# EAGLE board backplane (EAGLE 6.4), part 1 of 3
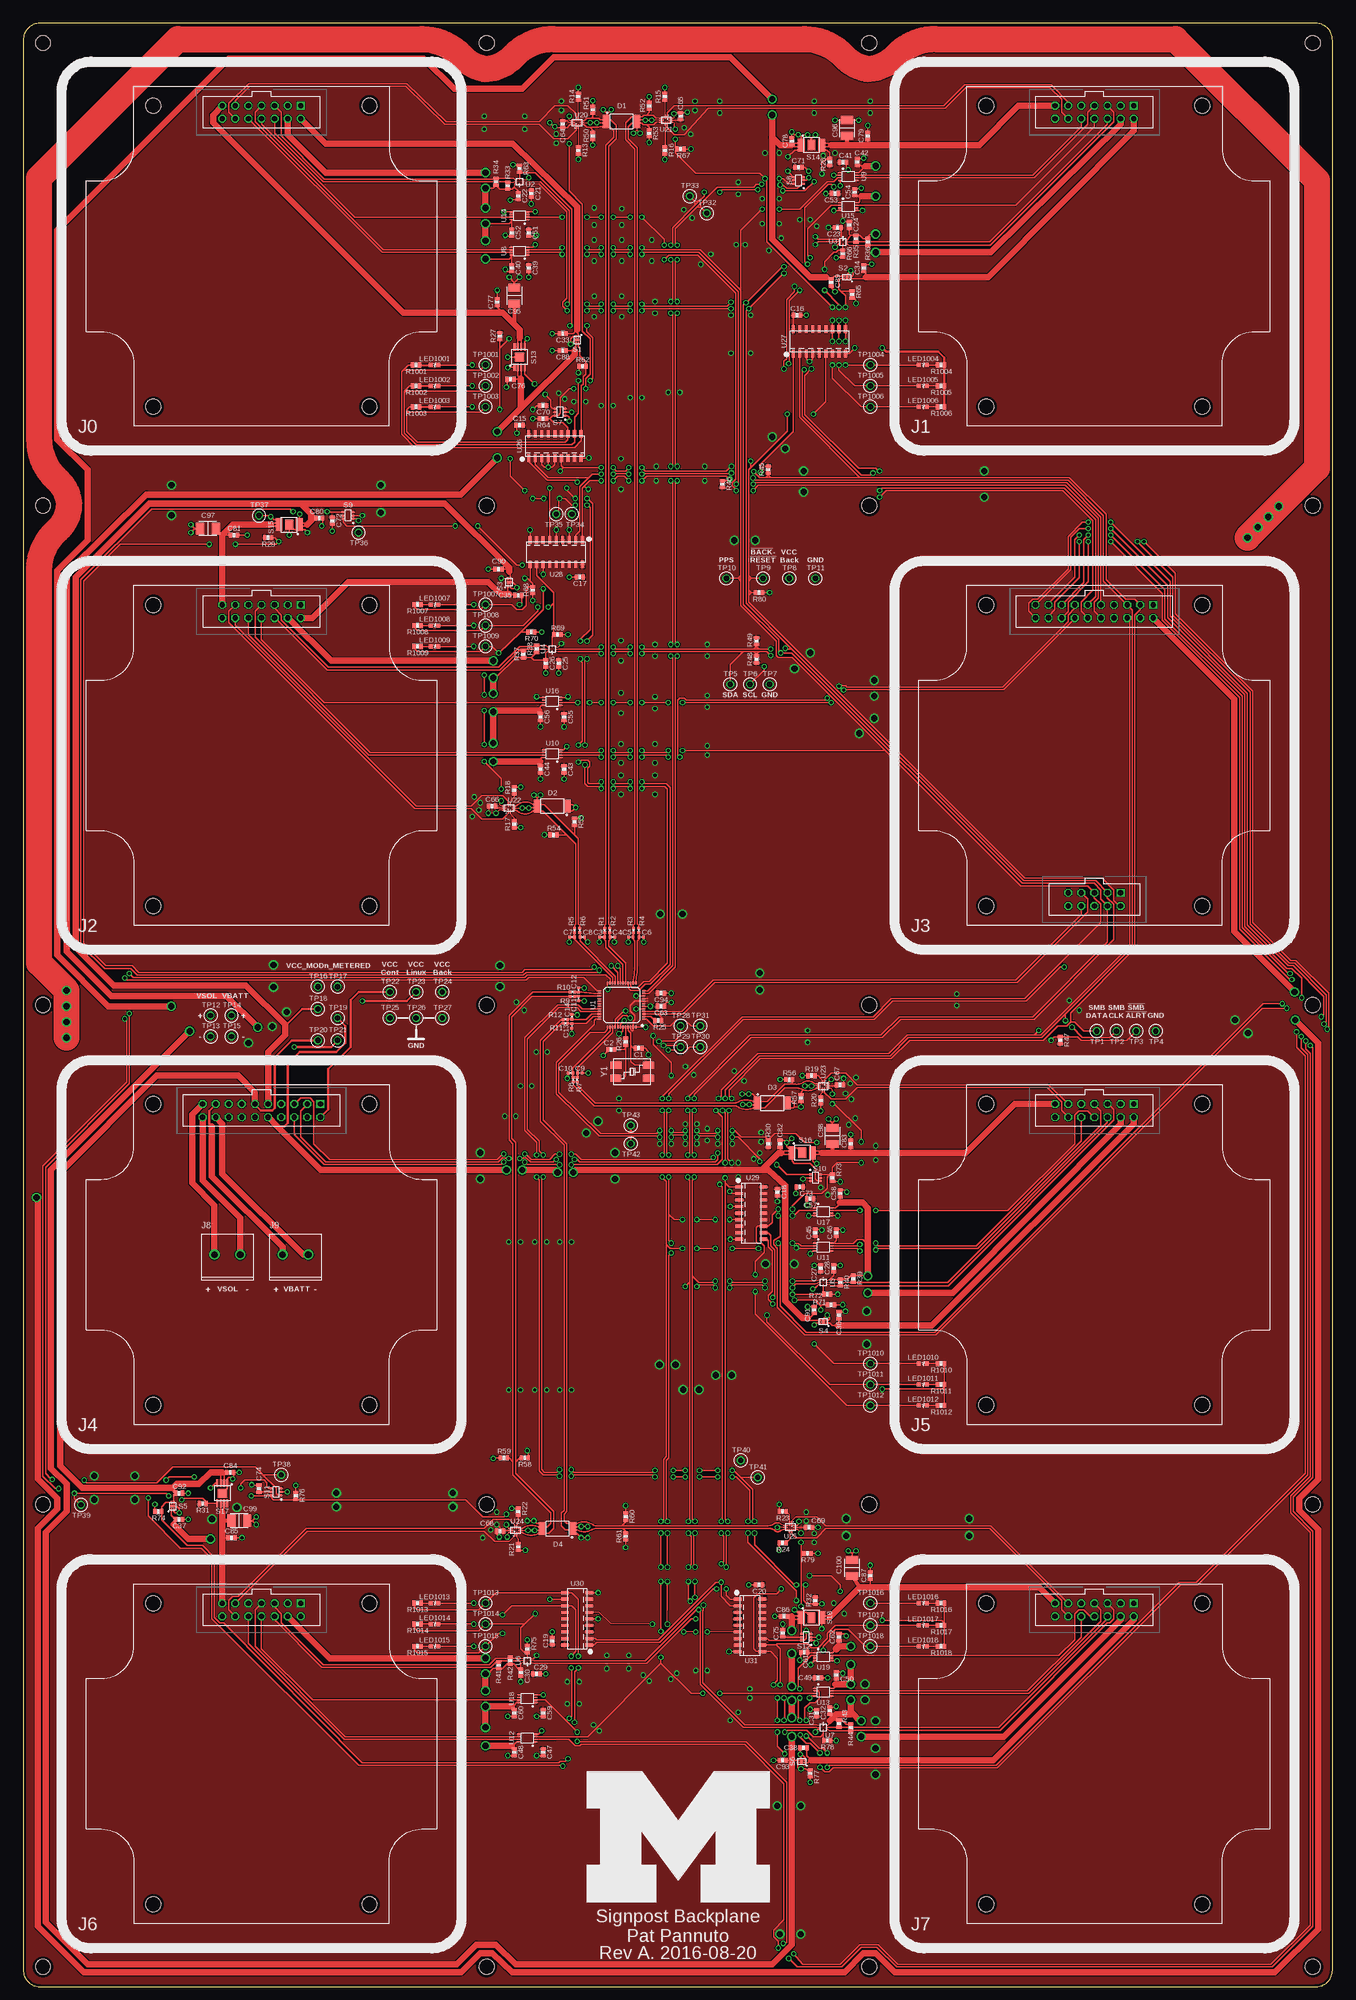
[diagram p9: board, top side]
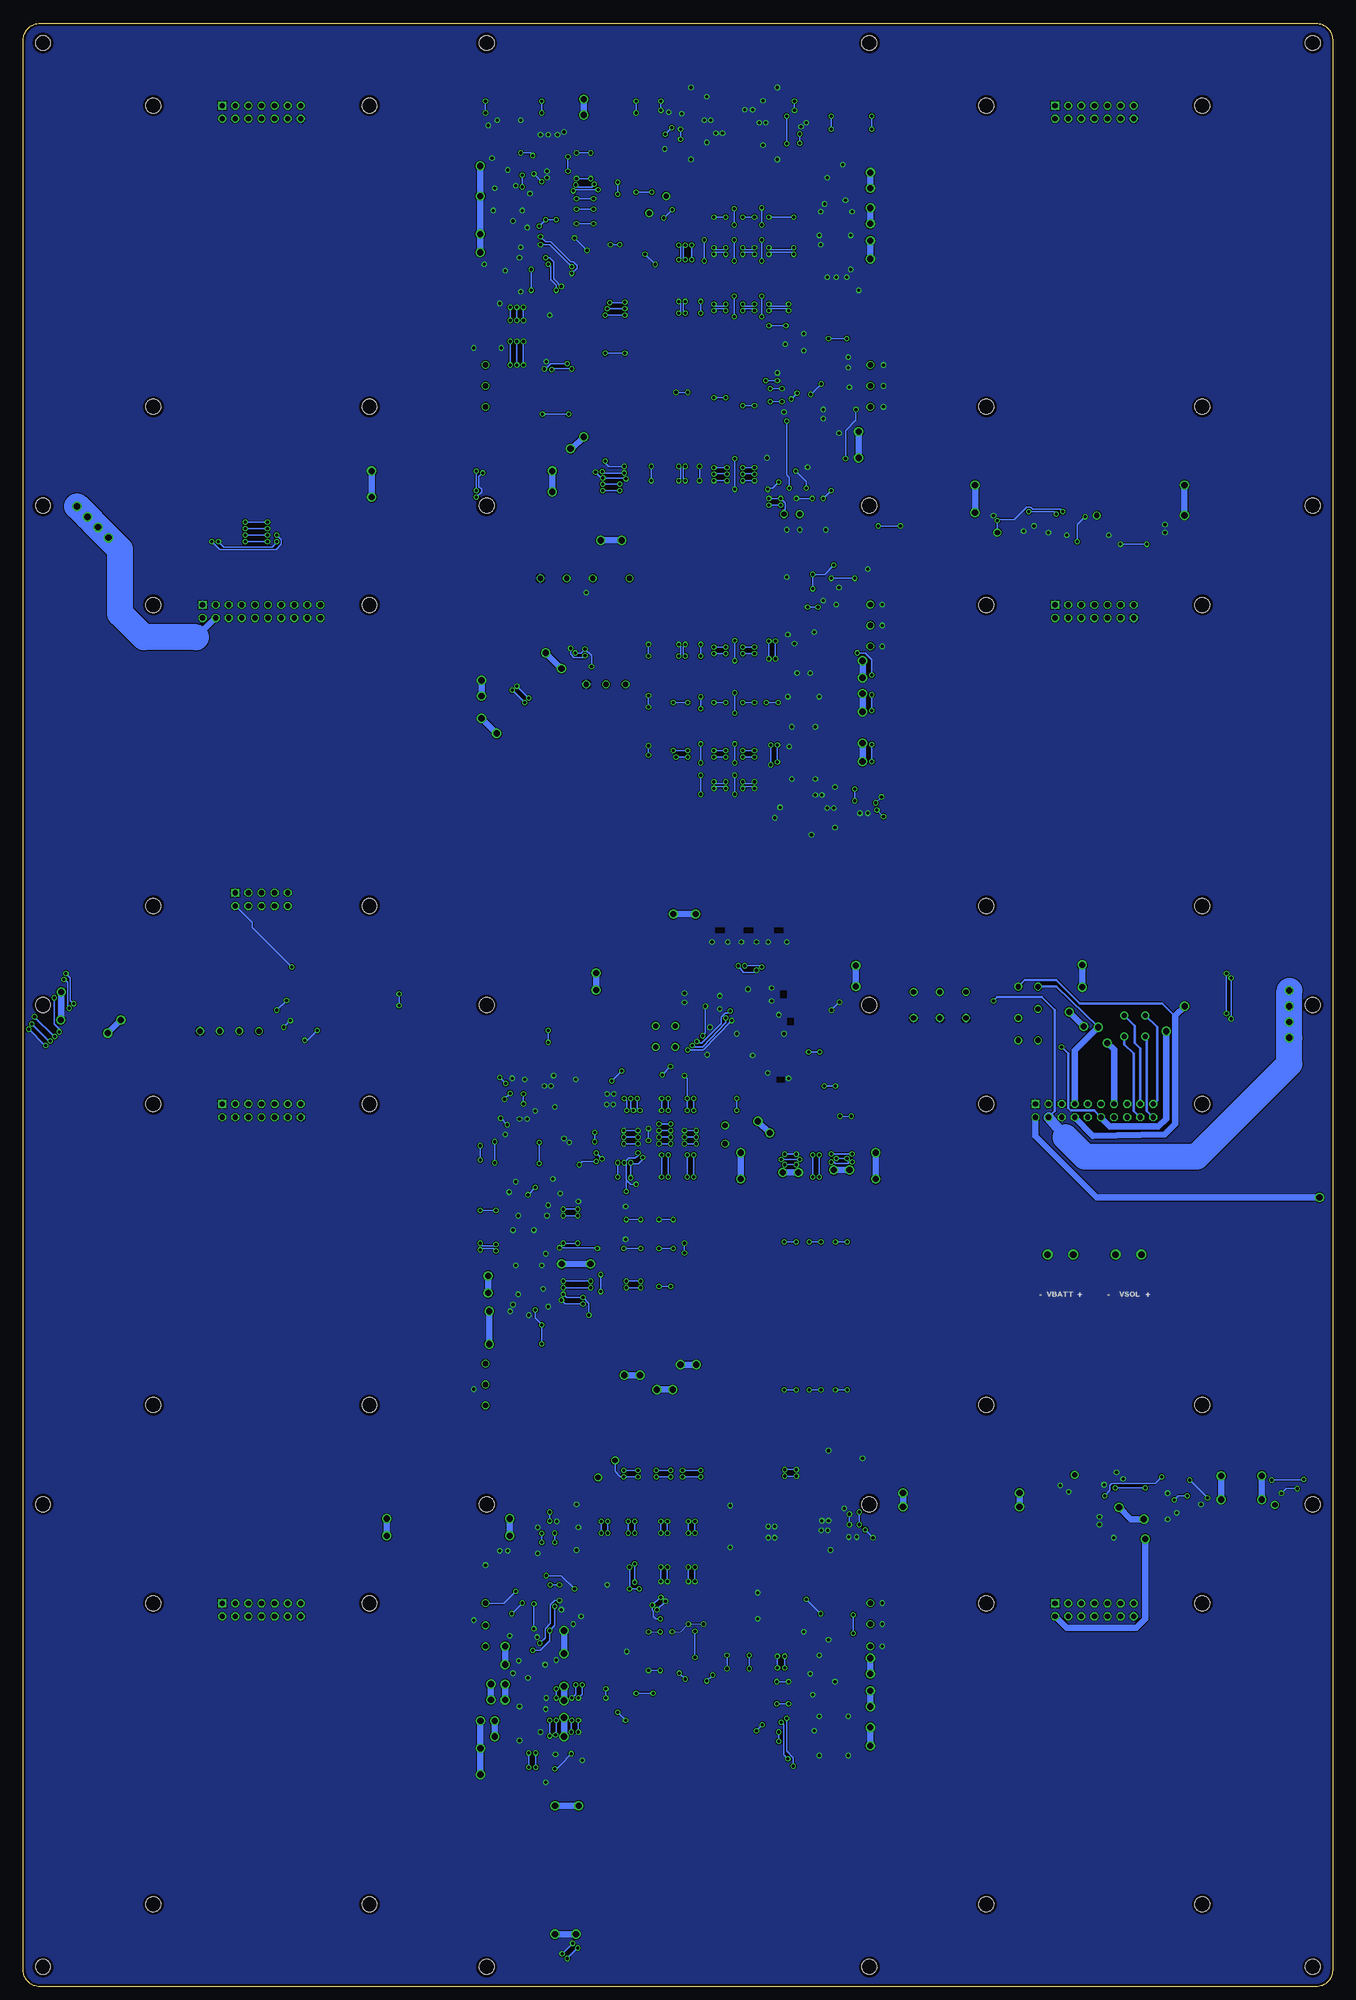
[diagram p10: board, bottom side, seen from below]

Size 254 x 381 mm. Coordinates in mm from the lower left corner, seen from the top.
Outline: 0,377.82 0,3.17 arc90 3.17,0 250.82,0 arc90 254,3.17 254,377.76 arc90 250.76,381 3.17,381 arc90 0,377.82
Copper layers (1*16): Top 0.0178mm / dielectric 59mil / Bottom 0.0178mm
Design rules "sunstone-2lyr_v1.0.0.3 *": minimum track width 6mil, minimum drill 14mil, track to track 6mil, track to pad 6mil, pad to pad 6mil, via to via 6mil, smd to smd 6mil, copper to edge 20mil, drill to drill 16mil, minimum pad ring 8mil, minimum via ring 8mil, stop-mask expansion 3mil, vias tented up to drill 50mil, thermal gap 10mil
Holes 2.95 mm at 3.81,3.81 250.19,3.81 250.19,377.19 3.81,377.19 89.87,377.19 164.13,377.19 3.81,287.38 89.87,287.38 164.13,287.38 250.19,287.38 3.81,190.5 89.87,190.5 164.13,190.5 250.19,190.5 3.81,93.62 89.87,93.62 164.13,93.62 250.19,93.62 89.87,3.81 164.13,3.81
tRestrict: area 120.2,191.5 to 120.5,191.5; area 118,186.1 to 118.1,186.4

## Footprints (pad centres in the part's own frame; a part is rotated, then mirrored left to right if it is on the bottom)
0603_CAP = smd 0.7 x 1: 1 -0.65,0; 2 0.65,0
0402_CAP = smd 0.536 x 0.546: 1 -0.433,0; 2 0.433,0
1210_CAP = smd 2.4 x 1.6: 1 0,1.55; 2 0,-1.55
TSSOP-8 = smd 1.5 x 0.45: 1 -2.9,0.975; 2 -2.9,0.325; 3 -2.9,-0.325; 4 -2.9,-0.975; 5 2.9,-0.975; 6 2.9,-0.325; 7 2.9,0.325; 8 2.9,0.975
BACKPLANE_MODULE_14PIN = drill 1.016 square: 1 7.62,29.21 | drill 1.016 octagon: 2 7.62,26.67; 3 5.08,29.21; 4 5.08,26.67; 5 2.54,29.21; 6 2.54,26.67; 7 0,29.21; 8 0,26.67; 9 -2.54,29.21; 10 -2.54,26.67; 11 -5.08,29.21; 12 -5.08,26.67; 13 -7.62,29.21; 14 -7.62,26.67 | hole 2.946: -20.955,29.21; 20.955,29.21; 20.955,-29.21; -20.955,-29.21
BACKPLANE_MODULE_20PIN_10PIN = drill 1.016 square: 1 11.43,29.21; 21 5.08,-26.67 | drill 1.016 octagon: 2 11.43,26.67; 3 8.89,29.21; 4 8.89,26.67; 5 6.35,29.21; 6 6.35,26.67; 7 3.81,29.21; 8 3.81,26.67; 9 1.27,29.21; 10 1.27,26.67; 11 -1.27,29.21; 12 -1.27,26.67; 13 -3.81,29.21; 14 -3.81,26.67; 15 -6.35,29.21; 16 -6.35,26.67; 17 -8.89,29.21; 18 -8.89,26.67; 19 -11.43,29.21; 20 -11.43,26.67; 22 5.08,-29.21; 23 2.54,-26.67; 24 2.54,-29.21; 25 0,-26.67; 26 0,-29.21; 27 -2.54,-26.67; 28 -2.54,-29.21; 29 -5.08,-26.67; 30 -5.08,-29.21 | hole 2.946: -20.955,29.21; 20.955,29.21; 20.955,-29.21; -20.955,-29.21
BACKPLANE_MODULE_20PIN = drill 1.016 square: 1 11.43,29.21 | drill 1.016 octagon: 2 11.43,26.67; 3 8.89,29.21; 4 8.89,26.67; 5 6.35,29.21; 6 6.35,26.67; 7 3.81,29.21; 8 3.81,26.67; 9 1.27,29.21; 10 1.27,26.67; 11 -1.27,29.21; 12 -1.27,26.67; 13 -3.81,29.21; 14 -3.81,26.67; 15 -6.35,29.21; 16 -6.35,26.67; 17 -8.89,29.21; 18 -8.89,26.67; 19 -11.43,29.21; 20 -11.43,26.67 | hole 2.946: -20.955,29.21; 20.955,29.21; 20.955,-29.21; -20.955,-29.21
PHEONIX-1935161 = drill 1.3: 1 0,0; 2 5,0
LED-0603 = smd 0.8 x 0.8: A 0,-0.75; C 0,0.75
0402_RES-HIGH_SPEED = smd 0.536 x 0.546: 1 -0.433,0; 2 0.433,0
0603-RES = smd 0.7 x 1: 1 -0.65,0; 2 0.65,0
TDFN4 = smd 0.3 x 0.55: 1 -0.25,-0.725; 2 0.25,-0.725; 3 0.25,0.725; 4 -0.25,0.725 | smd 0.86 x 0.5: PAD 0,0
SC70-6 = smd 0.4 x 0.5: 1 -0.65,-0.95; 2 0,-0.95; 3 0.65,-0.95; 4 0.65,0.95; 5 0,0.95; 6 -0.65,0.95
MSOP-8EP = smd 0.45 x 1.35: 1 -0.975,-1.975; 2 -0.325,-1.975; 3 0.325,-1.975; 4 0.975,-1.975; 5 0.975,1.975; 6 0.325,1.975; 7 -0.325,1.975; 8 -0.975,1.975 | smd 2 x 1.7: PAD 0,0
TESTPOINT_0.040IN = drill 1.016: TESTPOINT 0,0
LQFP-48 = smd 0.3 x 0.6: 1 -2.75,-4.3; 2 -2.25,-4.3; 3 -1.75,-4.3; 4 -1.25,-4.3; 5 -0.75,-4.3; 6 -0.25,-4.3; 7 0.25,-4.3; 8 0.75,-4.3; 9 1.25,-4.3; 10 1.75,-4.3; 11 2.25,-4.3; 12 2.75,-4.3; 25 2.75,4.3; 26 2.25,4.3; 27 1.75,4.3; 28 1.25,4.3; 29 0.75,4.3; 30 0.25,4.3; 31 -0.25,4.3; 32 -0.75,4.3; 33 -1.25,4.3; 34 -1.75,4.3; 35 -2.25,4.3; 36 -2.75,4.3 | smd 0.6 x 0.3: 13 4.3,-2.75; 14 4.3,-2.25; 15 4.3,-1.75; 16 4.3,-1.25; 17 4.3,-0.75; 18 4.3,-0.25; 19 4.3,0.25; 20 4.3,0.75; 21 4.3,1.25; 22 4.3,1.75; 23 4.3,2.25; 24 4.3,2.75; 37 -4.3,2.75; 38 -4.3,2.25; 39 -4.3,1.75; 40 -4.3,1.25; 41 -4.3,0.75; 42 -4.3,0.25; 43 -4.3,-0.25; 44 -4.3,-0.75; 45 -4.3,-1.25; 46 -4.3,-1.75; 47 -4.3,-2.25; 48 -4.3,-2.75
UMLP-8 = smd 0.35 x 0.25: 1 -0.55,0; 5 0.55,0 | smd 0.24 x 0.35: 2 -0.4,-0.625; 3 0,-0.625; 4 0.4,-0.625; 6 0.4,0.625; 7 0,0.625; 8 -0.4,0.625
VFSOP-8 = smd 0.25 x 0.75: 1 -0.75,-1.55; 2 -0.25,-1.55; 3 0.25,-1.55; 4 0.75,-1.55; 5 0.75,1.55; 6 0.25,1.55; 7 -0.25,1.55; 8 -0.75,1.55
UQFN-10 = smd 0.2 x 0.9: 1 -0.2,-0.65 | smd 0.2 x 0.8: 2 0.2,-0.7; 6 0.2,0.7; 7 -0.2,0.7 | smd 0.8 x 0.2: 3 0.9,-0.4; 4 0.9,0; 5 0.9,0.4; 8 -0.9,0.4; 9 -0.9,0; 10 -0.9,-0.4
SOIC-18 = smd 0.635 x 1.524: 1 -5.08,-2.362; 2 -3.81,-2.362; 3 -2.54,-2.362; 4 -1.27,-2.362; 5 0,-2.362; 6 1.27,-2.362; 7 2.54,-2.362; 8 3.81,-2.362; 9 5.08,-2.362; 10 5.08,2.362; 11 3.81,2.362; 12 2.54,2.362; 13 1.27,2.362; 14 0,2.362; 15 -1.27,2.362; 16 -2.54,2.362; 17 -3.81,2.362; 18 -5.08,2.362
ABMM = smd 2.21 x 1.397: 1 -3.167,-1.27; 3 3.15,1.27; NC1 -3.15,1.27; NC2 3.15,-1.27

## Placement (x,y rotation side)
C1  22pF, 5% tol  [0603_CAP]  119.38,182.12 180 top
C2  22pF, 5% tol  [0603_CAP]  114.05,181.86 0 top
C3  22pF  [0402_CAP]  112.27,203.71 180 top
C4  22pF  [0402_CAP]  114.3,203.71 0 top
C5  22pF  [0402_CAP]  117.86,203.71 180 top
C6  22pF  [0402_CAP]  119.89,203.71 0 top
C7  22pF  [0402_CAP]  106.43,203.71 180 top
C8  22pF  [0402_CAP]  108.46,203.71 0 top
C9  22pF  [0402_CAP]  107.95,177.29 0 top
C10  22pF  [0402_CAP]  106.17,177.29 180 top
C11  22pF  [0402_CAP]  107.7,191.77 270 top
C12  22pF  [0402_CAP]  107.7,193.42 90 top
C13  22pF  [0402_CAP]  106.43,186.44 270 top
C14  22pF  [0402_CAP]  106.43,188.21 90 top
C15  100nF  [0603_CAP]  96.27,303.02 180 top
C16  100nF  [0603_CAP]  150.11,324.36 0 top
C17  100nF  [0603_CAP]  107.95,273.56 180 top
C18  100nF  [0603_CAP]  146.3,154.18 270 top
C19  100nF  [0603_CAP]  102.62,67.06 90 top
C20  100nF  [0603_CAP]  142.75,77.98 180 top
C21  100nF  [0603_CAP]  98.55,347.98 270 top
C22  100nF  [0603_CAP]  96.01,347.47 270 top
C23  100nF  [0603_CAP]  157.99,341.38 180 top
C24  100nF  [0603_CAP]  160.27,341.88 90 top
C25  100nF  [0603_CAP]  103.89,256.79 270 top
C26  100nF  [0603_CAP]  101.35,256.79 270 top
C27  100nF  [0603_CAP]  154.69,139.45 90 top
C28  100nF  [0603_CAP]  157.23,139.45 90 top
C29  100nF  [0603_CAP]  99.57,60.71 0 top
C30  100nF  [0603_CAP]  96.52,60.96 270 top
C31  100nF  [0603_CAP]  153.92,53.09 90 top
C32  100nF  [0603_CAP]  156.46,53.59 90 top
C33  100nF  [0603_CAP]  104.65,320.8 180 top
C34  100nF  [0603_CAP]  163.07,333.5 90 top
C35  100nF  [0603_CAP]  96.01,270 0 top
C36  100nF  [0603_CAP]  158.24,130.3 90 top
C37  100nF  [0603_CAP]  30.23,90.68 0 top
C38  100nF  [0603_CAP]  151.38,46.35 180 top
C39  100nF  [0603_CAP]  98.04,333.5 270 top
C40  100nF  [0603_CAP]  94.74,333.5 270 top
C41  100nF  [0603_CAP]  159,354.08 0 top
C42  100nF  [0603_CAP]  161.8,354.08 90 top
C43  100nF  [0603_CAP]  104.9,236.22 270 top
C44  100nF  [0603_CAP]  100.33,236.22 270 top
C45  100nF  [0603_CAP]  153.67,146.3 90 top
C46  100nF  [0603_CAP]  157.73,146.3 90 top
C47  100nF  [0603_CAP]  100.84,45.47 270 top
C48  100nF  [0603_CAP]  95.25,45.47 270 top
C49  100nF  [0603_CAP]  154.18,59.94 0 top
C50  100nF  [0603_CAP]  157.73,60.45 90 top
C51  100nF  [0603_CAP]  98.04,340.36 270 top
C52  100nF  [0603_CAP]  94.74,340.36 270 top
C53  100nF  [0603_CAP]  157.48,347.98 180 top
C54  100nF  [0603_CAP]  161.29,348.23 90 top
C55  100nF  [0603_CAP]  104.9,246.38 270 top
C56  100nF  [0603_CAP]  100.33,246.38 270 top
C57  100nF  [0603_CAP]  152.65,152.91 180 top
C58  100nF  [0603_CAP]  158.5,153.92 90 top
C59  100nF  [0603_CAP]  100.84,53.09 270 top
C60  100nF  [0603_CAP]  95.25,53.09 270 top
C61  100nF  [0603_CAP]  151.51,64.9 180 top
C62  100nF  [0603_CAP]  158.24,67.82 90 top
C63  100nF  [0603_CAP]  123.7,190.25 180 top
C64  100nF  [0603_CAP]  104.65,361.44 90 top
C65  100nF  [0603_CAP]  127.51,362.97 270 top
C66  100nF  [0603_CAP]  90.93,229.11 0 top
C67  100nF  [0603_CAP]  158.47,175.01 180 top
C68  100nF  [0603_CAP]  92.46,88.39 0 top
C69  100nF  [0603_CAP]  152.4,89.15 180 top
C70  100nF  [0603_CAP]  100.84,306.83 180 top
C71  100nF  [0603_CAP]  150.37,353.06 0 top
C72  100nF  [0603_CAP]  59.94,284.48 270 top
C73  100nF  [0603_CAP]  150.62,155.19 180 top
C74  100nF  [0603_CAP]  45.72,96.65 90 top
C75  100nF  [0603_CAP]  147.32,68.58 90 top
C76  100nF  [0603_CAP]  94.49,311.91 180 top
C77  100nF  [0603_CAP]  91.95,326.9 90 top
C78  100nF  [0603_CAP]  149.1,358.14 90 top
C79  100nF  [0603_CAP]  163.83,359.16 90 top
C80  100nF  [0603_CAP]  57.4,284.99 0 top
C81  100nF  [0603_CAP]  40.89,281.69 0 top
C82  100nF  [0603_CAP]  146.81,163.58 90 top
C83  100nF  [0603_CAP]  160.53,163.58 90 top
C84  100nF  [0603_CAP]  40.13,99.82 0 top
C85  100nF  [0603_CAP]  40.39,87.12 0 top
C86  100nF  [0603_CAP]  147.57,71.88 180 top
C87  100nF  [0603_CAP]  164.34,79.76 90 top
C88  4.7uF  [0603_CAP]  104.65,317.5 180 top
C89  4.7uF  [0603_CAP]  156.72,330.71 270 top
C90  4.7uF  [0603_CAP]  92.2,275.08 180 top
C91  4.7uF  [0603_CAP]  153.42,131.32 90 top
C92  4.7uF  [0603_CAP]  30.23,95.76 0 top
C93  4.7uF  [0603_CAP]  147.32,43.94 180 top
C94  4.7uF  [0603_CAP]  123.7,192.79 180 top
C95  150uF  [1210_CAP]  95.25,328.17 180 top
C96  150uF  [1210_CAP]  159.77,360.68 180 top
C97  150uF  [1210_CAP]  35.81,282.96 270 top
C98  150uF  [1210_CAP]  156.97,165.1 180 top
C99  150uF  [1210_CAP]  41.91,90.42 90 top
C100  150uF  [1210_CAP]  160.78,81.28 180 top
D1  SN75240-TSSOP  [TSSOP-8]  116.08,361.95 0 top
D2  SN75240-TSSOP  [TSSOP-8]  102.62,229.11 180 top
D3  SN75240-TSSOP  [TSSOP-8]  145.29,171.45 0 top
D4  SN75240-TSSOP  [TSSOP-8]  103.63,88.9 180 top
J0  BACKPLANE_GENERIC_MODULE  [BACKPLANE_MODULE_14PIN]  46.2,335.81 0 top
J1  BACKPLANE_GENERIC_MODULE  [BACKPLANE_MODULE_14PIN]  207.8,335.81 0 top
J2  BACKPLANE_GENERIC_MODULE  [BACKPLANE_MODULE_14PIN]  46.2,238.94 0 top
J3  BACKPLANE_CONTROLLER_MODULE  [BACKPLANE_MODULE_20PIN_10PIN]  207.8,238.94 0 top
J4  BACKPLANE_POWER_MODULE  [BACKPLANE_MODULE_20PIN]  46.2,142.06 0 top
J5  BACKPLANE_GENERIC_MODULE  [BACKPLANE_MODULE_14PIN]  207.8,142.06 0 top
J6  BACKPLANE_GENERIC_MODULE  [BACKPLANE_MODULE_14PIN]  46.2,45.19 0 top
J7  BACKPLANE_GENERIC_MODULE  [BACKPLANE_MODULE_14PIN]  207.8,45.19 0 top
J8  SCREW_TERMINAL  [PHEONIX-1935161]  37.08,142.06 0 top
J9  SCREW_TERMINAL  [PHEONIX-1935161]  50.29,142.06 0 top
LED1001  LED0603  [LED-0603]  79.76,314.71 270 top
LED1002  LED0603  [LED-0603]  79.76,310.64 270 top
LED1003  LED0603  [LED-0603]  79.76,306.58 270 top
LED1004  LED0603  [LED-0603]  174.5,314.71 270 top
LED1005  LED0603  [LED-0603]  174.5,310.64 270 top
LED1006  LED0603  [LED-0603]  174.5,306.58 270 top
LED1007  LED0603  [LED-0603]  79.76,268.22 270 top
LED1008  LED0603  [LED-0603]  79.76,264.16 270 top
LED1009  LED0603  [LED-0603]  79.76,260.1 270 top
LED1010  LED0603  [LED-0603]  174.5,120.9 270 top
LED1011  LED0603  [LED-0603]  174.5,116.84 270 top
LED1012  LED0603  [LED-0603]  174.5,112.78 270 top
LED1013  LED0603  [LED-0603]  79.76,74.42 270 top
LED1014  LED0603  [LED-0603]  79.76,70.36 270 top
LED1015  LED0603  [LED-0603]  79.76,66.04 270 top
LED1016  LED0603  [LED-0603]  174.5,74.42 270 top
LED1017  LED0603  [LED-0603]  174.5,70.1 270 top
LED1018  LED0603  [LED-0603]  174.5,66.04 270 top
LOGO1  UMICH_SOLID_GIANT  [UMICH_SOLID_1000MIL]  109.35,16.38 0 top
R1  27Ω  [0402_RES-HIGH_SPEED]  112.78,204.98 90 top
R2  27Ω  [0402_RES-HIGH_SPEED]  113.79,204.98 90 top
R3  27Ω  [0402_RES-HIGH_SPEED]  118.36,204.98 90 top
R4  27Ω  [0402_RES-HIGH_SPEED]  119.38,204.98 90 top
R5  27Ω  [0402_RES-HIGH_SPEED]  106.93,204.98 90 top
R6  27Ω  [0402_RES-HIGH_SPEED]  107.95,204.98 90 top
R7  27Ω  [0402_RES-HIGH_SPEED]  107.44,176.02 270 top
R8  27Ω  [0402_RES-HIGH_SPEED]  106.68,176.02 270 top
R9  27Ω  [0402_RES-HIGH_SPEED]  106.55,192.15 180 top
R10  27Ω  [0402_RES-HIGH_SPEED]  106.55,193.04 180 top
R11  27Ω  [0402_RES-HIGH_SPEED]  105.16,186.94 180 top
R12  27Ω  [0402_RES-HIGH_SPEED]  105.16,187.71 180 top
R13  50Ω  [0603-RES]  107.7,356.36 270 top
R14  50Ω  [0603-RES]  107.7,366.78 90 top
R15  50Ω  [0603-RES]  124.46,366.78 90 top
R16  50Ω  [0603-RES]  124.46,356.36 270 top
R17  50Ω  [0603-RES]  95.25,225.55 270 top
R18  50Ω  [0603-RES]  95.25,232.16 90 top
R19  50Ω  [0603-RES]  152.91,176.78 180 top
R20  50Ω  [0603-RES]  154.69,171.96 270 top
R21  50Ω  [0603-RES]  96.01,85.34 270 top
R22  50Ω  [0603-RES]  96.01,92.2 90 top
R23  50Ω  [0603-RES]  147.32,92.2 180 top
R24  50Ω  [0603-RES]  147.32,86.11 180 top
R25  1.5kΩ  [0603-RES]  123.19,187.45 180 top
R26  1.5kΩ  [0603-RES]  116.84,183.39 90 top
R27  10kΩ  [0603-RES]  92.46,320.29 90 top
R28  10kΩ  [0603-RES]  156.46,354.08 270 top
R29  10kΩ  [0603-RES]  47.5,281.18 180 top
R30  10kΩ  [0603-RES]  144.53,163.58 270 top
R31  10kΩ  [0603-RES]  34.8,93.73 180 top
R32  10kΩ  [0603-RES]  153.67,74.93 90 top
R33  10kΩ  [0603-RES]  93.98,349.5 90 top
R34  10kΩ  [0603-RES]  91.69,350.27 90 top
R35  10kΩ  [0603-RES]  161.54,339.22 270 top
R36  10kΩ  [0603-RES]  163.83,338.58 270 top
R37  10kΩ  [0603-RES]  97.03,258.57 90 top
R38  10kΩ  [0603-RES]  99.57,259.59 90 top
R39  10kΩ  [0603-RES]  161.04,137.41 270 top
R40  10kΩ  [0603-RES]  158.5,136.65 270 top
R41  10kΩ  [0603-RES]  92.2,62.36 90 top
R42  10kΩ  [0603-RES]  94.49,63.25 90 top
R43  10kΩ  [0603-RES]  158.24,51.05 270 top
R44  10kΩ  [0603-RES]  160.53,50.29 270 top
R45  10kΩ  [0603-RES]  144.53,294.39 90 top
R46  10kΩ  [0603-RES]  135.64,291.59 270 top
R47  10kΩ  [0603-RES]  201.17,183.64 270 top
R48  10kΩ  [0603-RES]  142.24,257.56 270 top
R49  10kΩ  [0603-RES]  142.24,261.11 90 top
R50  15kΩ  [0603-RES]  110.49,359.16 90 top
R51  15kΩ  [0603-RES]  110.49,364.24 270 top
R52  15kΩ  [0603-RES]  121.41,365 270 top
R53  15kΩ  [0603-RES]  121.41,359.66 90 top
R54  15kΩ  [0603-RES]  102.87,223.52 0 top
R55  15kΩ  [0603-RES]  106.93,226.06 270 top
R56  15kΩ  [0603-RES]  148.59,176.02 0 top
R57  15kΩ  [0603-RES]  150.88,172.47 90 top
R58  15kΩ  [0603-RES]  97.28,102.62 180 top
R59  15kΩ  [0603-RES]  93.22,102.62 0 top
R60  15kΩ  [0603-RES]  116.84,91.19 270 top
R61  15kΩ  [0603-RES]  116.84,87.38 90 top
R62  10MΩ  [0603-RES]  108.46,314.45 0 top
R63  10MΩ  [0603-RES]  96.27,352.81 270 top
R64  10MΩ  [0603-RES]  100.84,304.29 0 top
R65  10MΩ  [0603-RES]  160.78,328.42 90 top
R66  10MΩ  [0603-RES]  159,336.3 90 top
R67  10MΩ  [0603-RES]  127.51,356.62 180 top
R68  10MΩ  [0603-RES]  98.81,271.02 90 top
R69  10MΩ  [0603-RES]  103.63,262.38 180 top
R70  10MΩ  [0603-RES]  98.55,262.89 180 top
R71  10MΩ  [0603-RES]  156.72,132.33 180 top
R72  10MΩ  [0603-RES]  155.96,134.37 180 top
R73  10MΩ  [0603-RES]  156.97,156.97 90 top
R74  10MΩ  [0603-RES]  26.16,92.2 0 top
R75  10MΩ  [0603-RES]  97.79,65.53 270 top
R76  10MΩ  [0603-RES]  52.83,95.25 270 top
R77  10MΩ  [0603-RES]  152.65,41.4 90 top
R78  10MΩ  [0603-RES]  155.96,47.75 180 top
R79  10MΩ  [0603-RES]  152.15,84.07 180 top
R80  10MΩ  [0603-RES]  142.75,270.51 180 top
R1001  15Ω  [0603-RES]  76.2,314.71 180 top
R1002  15Ω  [0603-RES]  76.2,310.64 180 top
R1003  15Ω  [0603-RES]  76.2,306.58 180 top
R1004  15Ω  [0603-RES]  178.05,314.71 180 top
R1005  15Ω  [0603-RES]  178.05,310.64 180 top
R1006  15Ω  [0603-RES]  178.05,306.58 180 top
R1007  15Ω  [0603-RES]  76.45,268.22 180 top
R1008  15Ω  [0603-RES]  76.45,264.16 180 top
R1009  15Ω  [0603-RES]  76.45,260.1 180 top
R1010  15Ω  [0603-RES]  178.05,120.9 180 top
R1011  15Ω  [0603-RES]  178.05,116.84 180 top
R1012  15Ω  [0603-RES]  178.05,112.78 180 top
R1013  15Ω  [0603-RES]  76.45,74.42 180 top
R1014  15Ω  [0603-RES]  76.45,70.36 180 top
R1015  15Ω  [0603-RES]  76.45,66.04 180 top
R1016  15Ω  [0603-RES]  178.05,74.42 180 top
R1017  15Ω  [0603-RES]  178.05,70.1 180 top
R1018  15Ω  [0603-RES]  178.05,66.04 180 top
S1  SIP3240X  [TDFN4]  107.44,319.53 180 top
S2  SIP3240X  [TDFN4]  159.77,331.72 90 top
S3  SIP3240X  [TDFN4]  94.23,272.54 0 top
S4  SIP3240X  [TDFN4]  155.19,129.03 90 top
S5  SIP3240X  [TDFN4]  28.96,93.22 0 top
S6  SIP3240X  [TDFN4]  151,43.69 90 top
S7  NC7SZ157  [SC70-6]  104.14,305.56 90 top
S8  NC7SZ157  [SC70-6]  150.37,350.52 90 top
S9  NC7SZ157  [SC70-6]  62.99,285.5 90 top
S10  NC7SZ157  [SC70-6]  153.67,156.97 270 top
S11  NC7SZ157  [SC70-6]  49.02,96.01 90 top
S12  NC7SZ157  [SC70-6]  151.89,67.82 90 top
S13  AP2401MP  [MSOP-8EP]  96.27,316.23 0 top
S14  AP2401MP  [MSOP-8EP]  152.91,357.38 270 top
S15  AP2401MP  [MSOP-8EP]  51.56,283.72 90 top
S16  AP2401MP  [MSOP-8EP]  151.13,161.8 270 top
S17  AP2401MP  [MSOP-8EP]  38.61,95.76 180 top
S18  AP2401MP  [MSOP-8EP]  152.91,71.63 270 top
TP1  TEST_POINT_0.040IN  [TESTPOINT_0.040IN]  208.28,185.42 0 top
TP2  TEST_POINT_0.040IN  [TESTPOINT_0.040IN]  212.09,185.42 0 top
TP3  TEST_POINT_0.040IN  [TESTPOINT_0.040IN]  215.9,185.42 0 top
TP4  TEST_POINT_0.040IN  [TESTPOINT_0.040IN]  219.71,185.42 0 top
TP5  TEST_POINT_0.040IN  [TESTPOINT_0.040IN]  137.16,252.73 0 top
TP6  TEST_POINT_0.040IN  [TESTPOINT_0.040IN]  140.97,252.73 0 top
TP7  TEST_POINT_0.040IN  [TESTPOINT_0.040IN]  144.78,252.73 0 top
TP8  TEST_POINT_0.040IN  [TESTPOINT_0.040IN]  148.59,273.3 0 top
TP9  TEST_POINT_0.040IN  [TESTPOINT_0.040IN]  143.51,273.3 0 top
TP10  TEST_POINT_0.040IN  [TESTPOINT_0.040IN]  136.4,273.3 0 top
TP11  TEST_POINT_0.040IN  [TESTPOINT_0.040IN]  153.67,273.3 0 top
TP12  TEST_POINT_0.040IN  [TESTPOINT_0.040IN]  36.32,188.47 0 top
TP13  TEST_POINT_0.040IN  [TESTPOINT_0.040IN]  36.32,184.4 0 top
TP14  TEST_POINT_0.040IN  [TESTPOINT_0.040IN]  40.39,188.47 0 top
TP15  TEST_POINT_0.040IN  [TESTPOINT_0.040IN]  40.39,184.4 0 top
TP16  TEST_POINT_0.040IN  [TESTPOINT_0.040IN]  57.15,194.06 0 top
TP17  TEST_POINT_0.040IN  [TESTPOINT_0.040IN]  60.96,194.06 0 top
TP18  TEST_POINT_0.040IN  [TESTPOINT_0.040IN]  57.15,189.74 0 top
TP19  TEST_POINT_0.040IN  [TESTPOINT_0.040IN]  60.96,187.96 0 top
TP20  TEST_POINT_0.040IN  [TESTPOINT_0.040IN]  57.15,183.64 0 top
TP21  TEST_POINT_0.040IN  [TESTPOINT_0.040IN]  60.96,183.64 0 top
TP22  TEST_POINT_0.040IN  [TESTPOINT_0.040IN]  71.12,193.04 0 top
TP23  TEST_POINT_0.040IN  [TESTPOINT_0.040IN]  76.2,193.04 0 top
TP24  TEST_POINT_0.040IN  [TESTPOINT_0.040IN]  81.28,193.04 0 top
TP25  TEST_POINT_0.040IN  [TESTPOINT_0.040IN]  71.12,187.96 0 top
TP26  TEST_POINT_0.040IN  [TESTPOINT_0.040IN]  76.2,187.96 0 top
TP27  TEST_POINT_0.040IN  [TESTPOINT_0.040IN]  81.28,187.96 0 top
TP28  TEST_POINT_0.040IN  [TESTPOINT_0.040IN]  127.51,186.44 0 top
TP29  TEST_POINT_0.040IN  [TESTPOINT_0.040IN]  127.51,182.37 0 top
TP30  TEST_POINT_0.040IN  [TESTPOINT_0.040IN]  131.32,182.37 0 top
TP31  TEST_POINT_0.040IN  [TESTPOINT_0.040IN]  131.32,186.44 0 top
TP32  TEST_POINT_0.040IN  [TESTPOINT_0.040IN]  132.59,344.17 0 top
TP33  TEST_POINT_0.040IN  [TESTPOINT_0.040IN]  129.29,347.47 0 top
TP34  TEST_POINT_0.040IN  [TESTPOINT_0.040IN]  106.43,285.75 0 top
TP35  TEST_POINT_0.040IN  [TESTPOINT_0.040IN]  103.38,285.75 0 top
TP36  TEST_POINT_0.040IN  [TESTPOINT_0.040IN]  65.02,282.19 180 top
TP37  TEST_POINT_0.040IN  [TESTPOINT_0.040IN]  45.72,285.5 0 top
TP38  TEST_POINT_0.040IN  [TESTPOINT_0.040IN]  50.04,99.31 0 top
TP39  TEST_POINT_0.040IN  [TESTPOINT_0.040IN]  11.18,93.47 180 top
TP40  TEST_POINT_0.040IN  [TESTPOINT_0.040IN]  139.19,102.11 0 top
TP41  TEST_POINT_0.040IN  [TESTPOINT_0.040IN]  142.49,98.81 0 top
TP42  TEST_POINT_0.040IN  [TESTPOINT_0.040IN]  117.86,163.58 180 top
TP43  TEST_POINT_0.040IN  [TESTPOINT_0.040IN]  117.86,167.13 0 top
TP1001  TEST_POINT_0.040IN  [TESTPOINT_0.040IN]  89.66,314.71 0 top
TP1002  TEST_POINT_0.040IN  [TESTPOINT_0.040IN]  89.66,310.64 0 top
TP1003  TEST_POINT_0.040IN  [TESTPOINT_0.040IN]  89.66,306.58 0 top
TP1004  TEST_POINT_0.040IN  [TESTPOINT_0.040IN]  164.34,314.71 0 top
TP1005  TEST_POINT_0.040IN  [TESTPOINT_0.040IN]  164.34,310.64 0 top
TP1006  TEST_POINT_0.040IN  [TESTPOINT_0.040IN]  164.34,306.58 0 top
TP1007  TEST_POINT_0.040IN  [TESTPOINT_0.040IN]  89.66,268.22 0 top
TP1008  TEST_POINT_0.040IN  [TESTPOINT_0.040IN]  89.66,264.16 0 top
TP1009  TEST_POINT_0.040IN  [TESTPOINT_0.040IN]  89.66,260.1 0 top
TP1010  TEST_POINT_0.040IN  [TESTPOINT_0.040IN]  164.34,120.9 0 top
TP1011  TEST_POINT_0.040IN  [TESTPOINT_0.040IN]  164.34,116.84 0 top
TP1012  TEST_POINT_0.040IN  [TESTPOINT_0.040IN]  164.34,112.78 0 top
TP1013  TEST_POINT_0.040IN  [TESTPOINT_0.040IN]  89.66,74.42 0 top
TP1014  TEST_POINT_0.040IN  [TESTPOINT_0.040IN]  89.66,70.36 0 top
TP1015  TEST_POINT_0.040IN  [TESTPOINT_0.040IN]  89.66,66.04 0 top
TP1016  TEST_POINT_0.040IN  [TESTPOINT_0.040IN]  164.34,74.42 0 top
TP1017  TEST_POINT_0.040IN  [TESTPOINT_0.040IN]  164.34,70.1 0 top
TP1018  TEST_POINT_0.040IN  [TESTPOINT_0.040IN]  164.34,66.04 0 top
U1  TUSB2077A  [LQFP-48]  116.08,190.5 90 top
U2  FXMA2102  [UMLP-8]  96.27,350.27 90 top
U3  FXMA2102  [UMLP-8]  159,338.58 270 top
U4  FXMA2102  [UMLP-8]  102.62,259.59 90 top
U5  FXMA2102  [UMLP-8]  155.19,136.65 270 top
U6  FXMA2102  [UMLP-8]  97.79,63.25 90 top
U7  FXMA2102  [UMLP-8]  155.19,50.29 270 top
U8  SN74LVC2T45  [VFSOP-8]  96.27,336.8 90 top
U9  SN74LVC2T45  [VFSOP-8]  160.02,351.28 270 top
U10  SN74LVC2T45  [VFSOP-8]  102.62,239.27 90 top
U11  SN74LVC2T45  [VFSOP-8]  155.19,143.51 270 top
U12  SN74LVC2T45  [VFSOP-8]  97.79,48.26 90 top
U13  SN74LVC2T45  [VFSOP-8]  155.19,57.15 270 top
U14  SN74LVC2T45  [VFSOP-8]  96.27,343.66 90 top
U15  SN74LVC2T45  [VFSOP-8]  160.02,345.44 270 top
U16  SN74LVC2T45  [VFSOP-8]  102.62,249.43 90 top
U17  SN74LVC2T45  [VFSOP-8]  155.19,150.37 270 top
U18  SN74LVC2T45  [VFSOP-8]  97.79,55.88 90 top
U19  SN74LVC2T45  [VFSOP-8]  155.19,64.01 270 top
U20  TS3USB30E  [UQFN-10]  107.44,361.7 0 top
U21  TS3USB30E  [UQFN-10]  124.71,362.2 180 top
U22  TS3USB30E  [UQFN-10]  94.23,228.73 0 top
U23  TS3USB30E  [UQFN-10]  155.19,174.75 180 top
U24  TS3USB30E  [UQFN-10]  95.5,88.52 0 top
U25  TS3USB30E  [UQFN-10]  148.84,89.15 180 top
U26  MCP23008  [SOIC-18]  103.12,298.96 0 top
U27  MCP23008  [SOIC-18]  154.43,319.28 0 top
U28  MCP23008  [SOIC-18]  103.38,278.38 180 top
U29  MCP23008  [SOIC-18]  141.22,150.11 270 top
U30  MCP23008  [SOIC-18]  107.44,71.37 90 top
U31  MCP23008  [SOIC-18]  140.97,70.1 270 top
Y1  ABMM  [ABMM]  118.11,177.55 0 top

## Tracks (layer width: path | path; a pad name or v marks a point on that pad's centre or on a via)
!BACKPLANE_RESET  (via drill 0.6)
  Top 0.203: U31.6 v132.72,68.83 | v130.43,68.83 v128.14,68.83 | v124.97,70.36 124.97,73.03 | v122.05,70.36 114.05,70.36 111.76,72.64 U30.6
  Top 0.254: J3.22 212.67,209.73 211.58,210.82 211.58,212.85 209.3,215.14 194.31,215.14 140.72,268.73 140.72,270 | v201.93,197.87 201.17,197.87 194.56,191.26 168.66,191.26 165.1,187.71 139.7,187.71 125.22,173.23 v125.22,172.34 | v125.22,170.05 124.84,169.67 124.84,161.8 v125.22,161.42 | v125.22,157.1 125.22,149.86 | 125.22,149.86 126.24,148.84 v127.89,148.84 | v130.68,148.84 v134.24,148.84 | v137.03,148.84 U29.6 | 125.22,149.86 125.22,144.78 v125.73,144.27 | v125.73,142.37 125.22,141.86 125.22,102.62 124.71,102.11 124.71,90.55 v124.97,90.3 | v124.97,88.01 v124.97,81.41 | v124.97,78.61 124.97,73.03 | 140.72,270 140.72,271.02 | 140.72,271.02 140.72,272.8 | 140.72,272.8 140.72,273.81 | 140.72,273.81 140.72,294.39 141.1,294.77 | 141.1,294.77 148.21,301.88 v148.21,305.18 | v153.29,305.18 155.7,307.59 U27.6 | 141.1,294.77 v141.1,296.04 | v137.39,295.02 137.29,295.02 136.4,294.13 120.65,294.13 v120.02,294.77 | v117.47,294.77 116.84,294.13 115.06,294.13 v114.43,294.77 | v112.14,294.77 104.78,294.77 | 104.78,294.77 104.39,295.15 U26.6 | U28.6 v102.11,290.83 | v104.14,294.13 104.78,294.77 | R80.2 141.22,270.51 | 141.22,270.51 140.72,270 | 141.22,270.51 140.72,271.02 | v125.73,176.78 125.73,179.32 122.17,182.88 v122.17,184.53 | v121.67,190.25 U1.6 | TP9.TESTPOINT 141.22,273.3 | 141.22,273.3 140.72,272.8 | 141.22,273.3 140.72,273.81
  Bottom 0.203: v132.72,68.83 v130.43,68.83 | v128.14,68.83 126.49,68.83 v124.97,70.36 v122.05,70.36
  Bottom 0.254: J3.22 212.78,209.73 209.55,206.5 209.55,205.49 v201.93,197.87 | v125.22,170.05 v125.22,172.34 125.22,176.28 v125.73,176.78 | v125.22,161.42 v125.22,157.1 | v127.89,148.84 v130.68,148.84 | v134.24,148.84 v137.03,148.84 | v125.73,144.27 v125.73,142.37 | v124.97,90.3 v124.97,88.01 | v124.97,81.41 v124.97,78.61 | v148.21,305.18 v153.29,305.18 | v141.1,296.04 141.1,295.66 140.46,295.02 v137.39,295.02 | v120.02,294.77 v117.47,294.77 | v114.43,294.77 v112.14,294.77 | v102.11,290.83 102.11,292.1 v104.14,294.13 | v121.67,190.25 121.67,185.04 v122.17,184.53
!SMBALERT  (via drill 0.6)
  Top 0.254: J3.6 214.2,265.61 214.63,265.18 214.63,201.93 197.36,184.66 196.09,184.66 | 196.09,184.66 171.45,184.66 167.89,181.1 142.49,181.1 135.38,173.99 135.38,172.85 v134.87,172.34 | v93.22,160.02 92.71,159.51 58.42,159.51 52.58,165.35 52.58,168.71 J4.6 | v106.3,159.51 134.62,159.51 135.64,160.53 135.64,168.78 v134.37,170.05 | v97.28,160 97.77,159.51 v104.01,159.51 | 196.09,184.66 v196.98,185.55 | v199.39,183.64 200.04,184.29 R47.1 204.58,184.29 205.23,183.64 214.12,183.64 TP3.TESTPOINT
  Bottom 0.254: v134.87,172.34 134.87,170.56 v134.37,170.05 | v93.22,160.02 93.83,160.02 94.08,159.77 96.47,159.77 96.7,160 v97.28,160 | v106.3,159.51 v104.01,159.51 | v196.98,185.55 198.88,183.64 v199.39,183.64
CONT_MOD0_IN  (via drill 0.6)
  Top 0.254: J3.9 209.07,285.22 202.44,291.85 141.86,291.85 v141.6,291.59 | v138.3,291.59 138.68,291.97 138.68,328.93 131.06,336.55 120.4,336.55 v120.02,336.17 | U8.2 104.14,336.55 v104.52,336.17 | v109.35,336.17 109.73,336.55 111.76,336.55 v112.14,336.17 | v114.43,336.17 114.81,336.55 117.35,336.55 v117.73,336.17
  Bottom 0.254: v141.6,291.59 v138.3,291.59 | v104.52,336.17 104.9,336.55 108.97,336.55 v109.35,336.17 | v112.14,336.17 112.52,336.55 114.05,336.55 v114.43,336.17 | v117.73,336.17 118.11,336.55 119.63,336.55 v120.02,336.17
CONT_MOD0_OUT  (via drill 0.6)
  Top 0.254: J3.10 209.07,265.66 207.77,266.95 207.77,268.73 208.53,269.49 208.53,284.99 202.18,291.34 142.62,291.34 v141.6,290.32 | v138.3,290.32 138.3,290.47 137.49,291.29 137.49,291.9 138.18,292.58 138.18,328.68 130.81,336.04 125.22,336.04 v124.33,335.15 | v109.35,343.41 v112.14,343.41 | v114.43,343.41 v117.73,343.41 | v104.52,343.41 U14.2 | v124.33,337.95 124.33,339.09 v120.02,343.41
  Bottom 0.254: v141.6,290.32 v138.3,290.32 | v104.52,343.41 v109.35,343.41 | v112.14,343.41 v114.43,343.41 | v117.73,343.41 v120.02,343.41 | v124.33,335.15 v124.33,337.95
CONT_MOD1_IN  (via drill 0.6)
  Top 0.254: J3.11 206.53,268.25 208.03,269.75 208.05,284.71 201.93,290.83 166.62,290.83 v166.12,290.32 | v148.46,314.96 148.59,315.09 148.59,327.15 v150.62,329.18 | v152.15,334.26 151.64,334.77 151.64,345.19 156.21,349.76 156.72,349.76 v157.23,349.25 | U9.2 v157.23,351.54 | v166.12,294.13 165.86,294.13 165.35,294.64 162.05,294.64 151.64,305.05 151.64,312.67 v152.91,313.94
  Bottom 0.254: v166.12,290.32 v166.12,294.13 | v150.62,329.18 150.62,330.2 151.64,331.22 151.64,333.76 v152.15,334.26 | v157.23,349.25 v157.23,351.54 | v152.91,313.94 152.65,313.94 151.64,314.96 v148.46,314.96
CONT_MOD1_OUT  (via drill 0.6)
  Top 0.254: J3.12 206.53,265.66 205.23,266.95 205.23,268.73 207.52,271.02 207.52,284.48 201.68,290.32 167.39,290.32 v166.12,289.05 | v149.61,329.95 149.61,328.93 148.08,327.41 148.08,315.98 147.57,315.47 v147.57,313.94 | v152.65,335.53 152.15,336.04 152.15,341.12 156.71,345.69 U15.2 | v164.85,293.75 164.72,293.75 164.34,293.37 162.56,293.37 151.13,304.8 151.13,313.44 v151.51,313.82
  Bottom 0.254: v166.12,289.05 165.1,290.07 165.1,290.58 165.61,291.08 165.61,292.99 v164.85,293.75 | v149.61,329.95 151.13,331.47 151.13,334.77 151.89,335.53 v152.65,335.53 | v151.51,313.82 151.38,313.94 v147.57,313.94
CONT_MOD2_IN  (via drill 0.6)
  Top 0.254: J3.13 203.99,267.49 202.69,266.19 202.69,264.92 189.99,252.22 159.77,252.22 159.51,252.48 158.37,252.48 v158.24,252.35 | U10.2 111.76,239.02 v112.14,238.63 | v114.43,238.63 114.81,239.01 117.35,239.01 v117.73,238.63 | v120.02,238.63 120.4,239.01 124.71,239.01 v125.09,238.63 | v127.38,238.63 127,239.01 127,249.68 127.38,250.06 128.27,250.06 128.65,249.68 155.57,249.68 v155.96,250.06
  Bottom 0.254: v112.14,238.63 v114.43,238.63 | v117.73,238.63 v120.02,238.63 | v125.09,238.63 v127.38,238.63 | v155.96,250.06 v158.24,252.35
CONT_MOD2_OUT  (via drill 0.6)
  Top 0.254: J3.14 203.99,265.45 190.25,251.71 159.26,251.71 v159.13,251.59 | v112.14,249.18 v112.14,249.17 v109.86,249.17 | v114.43,249.17 v117.73,249.17 | v120.02,249.17 v125.09,249.17 | v127.89,249.17 v156.72,249.17 | U16.2 v107.56,249.18 v107.57,249.17
  Bottom 0.254: v112.14,249.17 v114.43,249.17 | v117.73,249.17 v120.02,249.17 | v125.09,249.17 v127.89,249.17 | v156.72,249.17 v159.13,251.59 | v107.57,249.17 v109.86,249.17
CONT_MOD5_IN  (via drill 0.6)
  Top 0.254: J3.15 205.74,272.44 205.74,280.8 v206.63,281.69 | v210.95,281.69 221.49,271.14 221.49,265.43 236.47,250.44 236.47,205.49 245.36,196.6 v245.75,196.6 | v244.22,190.75 240.54,190.75 176.78,127 151.89,127 146.81,132.08 146.81,143.89 v146.43,144.27 | U11.2 150.88,143.76 150.37,144.27 v149.22,144.27
  Bottom 0.254: v206.63,281.69 v210.95,281.69 | v245.75,196.6 244.86,195.71 244.86,191.39 v244.22,190.75 | v146.43,144.27 v149.22,144.27
CONT_MOD5_OUT  (via drill 0.6)
  Top 0.254: J3.16 202.69,266.85 202.69,268.73 206.63,272.67 v206.63,280.42 | v210.95,280.42 220.98,270.38 220.98,265.18 235.97,250.19 235.97,205.23 245.75,195.45 v246.13,195.45 | v245.11,189.87 240.41,189.87 177.04,126.49 151.64,126.49 146.3,131.83 146.3,143.26 145.54,144.02 145.54,144.78 146.81,145.54 146.81,149.22 v146.43,149.61 | v149.22,149.61 149.48,149.61 150.5,150.62 U17.2
  Bottom 0.254: v206.63,280.42 v210.95,280.42 | v246.13,195.45 245.36,194.82 245.36,190.12 v245.11,189.87 | v146.43,149.61 v149.22,149.61
CONT_MOD6_IN  (via drill 0.6)
  Top 0.254: U12.2 103.37,48.01 103.38,48.01 105.79,48.01 107.06,46.74 107.95,46.74 108.2,46.99 139.95,46.99 147.57,39.37 147.57,12.95 145.54,10.92 145.54,9.65 146.43,8.76 v146.43,7.49 | v148.46,5.46 150.11,3.81 158.75,3.81 162.56,7.62 165.61,7.62 169.42,3.81 242.32,3.81 250.19,11.68 250.19,88.39 246.38,92.2 246.38,95 250.19,98.81 250.19,182.12 v249.68,182.63 | v252.98,185.8 253.24,186.06 253.24,192.79 246.89,199.14 245.87,199.14 238.51,206.5 238.51,251.46 223.52,266.45 223.52,274.32 v217.42,280.42 | J3.17 198.91,268.5 203.96,273.56 203.96,280.8 v204.85,281.69
  Bottom 0.254: v146.43,7.49 v148.46,5.46 | v249.68,182.63 249.81,182.63 v252.98,185.8 | v204.85,281.69 203.96,280.8 203.96,279.91 204.98,278.89 215.9,278.89 v217.42,280.42
CONT_MOD6_OUT  (via drill 0.6)
  Top 0.254: U18.2 101.22,55.63 v107.44,49.4 | v149.48,6.35 151.26,4.32 158.5,4.32 162.31,8.13 165.86,8.13 169.67,4.32 242.06,4.32 249.68,11.94 249.68,88.14 245.87,91.95 245.87,95.25 249.68,99.06 249.68,181.1 248.79,181.99 v248.79,183.51 | v252.35,186.82 252.78,187.25 252.78,192.48 246.63,198.63 245.62,198.63 238,206.25 238,251.21 223.01,266.19 223.01,273.56 v216.15,280.42 | J3.18 198.91,265.96 200.15,267.21 200.15,268.73 204.85,273.43 v204.85,280.42 | v147.45,8.38 147.83,8.38 148.08,8.64 148.08,39.62 140.21,47.5 107.57,47.5 v107.44,47.62
  Bottom 0.254: v107.44,49.4 v107.44,47.62 | v147.45,8.38 v149.48,6.35 | v248.79,183.51 249.05,183.51 v252.35,186.82 | v204.85,280.42 204.85,280.29 205.74,279.4 215.14,279.4 v216.15,280.42
CONT_MOD7_IN  (via drill 0.6)
  Top 0.254: v210.95,282.96 222,271.91 222,265.68 236.98,250.7 236.98,205.74 245.11,197.61 246.13,197.61 248.03,195.71 v248.03,191.9 | U13.2 154.18,57.4 154.43,57.15 154.43,55.88 153.67,55.12 152.65,55.12 151.64,54.1 151.64,51.94 v151.89,51.69 | v151.89,48.64 152.02,48.64 154.43,46.23 155.07,46.23 v155.96,45.34 | v155.96,42.55 156.34,42.93 188.72,42.93 224.28,78.49 227.58,78.49 248.67,99.57 248.67,180.59 247.01,182.25 v247.01,185.29 | v206.63,282.96 204.85,282.96 203.2,281.31 203.2,274.98 J3.19
  Bottom 0.254: v151.89,51.69 v151.89,48.64 | v155.96,45.34 v155.96,42.55 | v247.01,185.29 247.01,185.8 248.03,186.82 v248.03,191.9 | v210.95,282.96 v206.63,282.96
CONT_MOD7_OUT  (via drill 0.6)
  Top 0.254: v210.95,284.23 222.5,272.67 222.5,265.94 237.49,250.95 237.49,205.99 245.36,198.12 246.38,198.12 252.32,192.18 252.32,188.7 v251.84,188.21 | U19.2 152.9,64.26 150.37,61.72 150.37,58.04 v150.62,57.78 | v150.62,56.01 150.62,55.88 150.37,55.63 150.37,51.94 v150.62,51.69 | v150.75,48.9 150.75,48.39 151.89,47.24 152.65,47.24 v154.56,45.34 | v154.56,42.55 155.45,41.66 156.34,41.66 157.1,42.42 188.98,42.42 224.54,77.98 227.84,77.98 249.17,99.31 249.17,180.85 247.9,182.12 v247.9,184.4 | v206.63,284.23 205.49,284.23 202.69,281.43 202.69,275.08 196.85,269.24 195.83,269.24 195.07,268.48 195.07,266.9 J3.20
  Bottom 0.254: v150.62,57.78 v150.62,56.01 | v150.62,51.69 150.62,49.02 v150.75,48.9 | v154.56,45.34 v154.56,42.55 | v247.9,184.4 248.03,184.4 v251.84,188.21 | v210.95,284.23 v206.63,284.23
CONT_USB+
  Top 0.254: 123.19,188.72 121.41,188.72 121.38,188.75 U1.3 | 123.19,188.72 128.02,188.72 134.11,194.82 192.79,194.82 206.5,208.53 206.5,211.02 J3.27 | R25.1 123.84,188.07 123.19,188.72
CONT_USB-
  Top 0.254: U1.4 121.18,189.25 121.41,189.23 127.76,189.23 133.86,195.33 192.53,195.33 205.26,208.05 J3.28
GND  (via drill 0.6)
  Top 0.203: U20.10 106.03,361.3 | U20.4 v109.98,361.7 v111.25,361.7 112.01,361.7 112.08,361.62 D1.3 | U21.4 v121.92,362.2 | D1.5 118.98,360.32 | 118.98,360.32 v119.63,359.66 | 118.98,360.32 118.98,360.28 v118.36,359.66 | U21.10 126.13,362.6 126.24,362.71 v126.24,363.47 | U3.4 158.1,338.18 | U25.4 v146.3,89.15 | U24.4 v97.92,88.52 | U7.4 154.16,49.89 | U5.4 154.29,136.25 154.05,136.02 | U23.10 156.09,175.4 | v152.91,174.75 U23.4 v151.64,174.75 | U25.10 150.26,89.55 150.37,89.66 | U6.4 98.95,63.65 | U24.10 94.22,88.12 93.85,87.76 v93.85,87.25 | U22.4 v96.77,228.73 | C66.1 90.28,227.82 v90.17,227.71 v91.69,227.71 92.31,228.33 U22.10 | U4.4 103.78,259.99 v104.39,260.6 | U2.4 97.68,350.67 v98.04,351.03
  Top 0.254: 106.03,361.3 105.52,360.79 C64.1 103.27,360.79 v103.12,360.93 102.87,360.93 v102.11,361.7 | D1.1 113.18,363.58 | 113.18,363.58 v112.52,364.24 | 113.18,363.58 113.39,363.58 v114.05,364.24 | D1.7 120.58,362.27 v120.65,362.2 v121.92,362.2 | v126.24,363.47 126.38,363.62 C65.1 128.67,363.62 v128.78,363.73 | C78.2 v149.1,359.92 149.61,359.41 v150.37,359.41 150.88,358.9 | S14.1 150.93,358.85 150.88,358.9 | 150.88,358.9 151.38,359.41 v152.15,359.41 152.91,358.65 | S14.PAD 152.91,358.65 | v153.67,359.41 152.91,358.65 | C42.2 162.96,354.73 v163.07,354.84 | C79.2 v163.83,361.19 | C53.2 v155.7,347.98 | C54.2 162.45,348.88 v162.56,349 | U9.4 158.47,349.53 v158.5,349.5 | C23.2 v156.21,341.38 | U15.4 v157.24,344.69 v157.23,344.68 | U15.5 v162.8,344.69 v162.81,344.68 | C34.2 164.48,334.15 v164.59,334.26 | R66.1 157.88,335.65 v157.73,335.53 | 158.1,338.18 v157.48,337.57 | C16.2 v151.89,324.36 | R13.2 v107.7,354.58 | R14.2 v107.7,368.55 | R50.1 v110.49,357.38 | R51.1 v110.49,366.01 | R16.2 v124.46,354.58 | R15.2 v124.46,368.55 | R53.1 v121.41,357.89 | R52.1 v121.41,366.78 | R57.1 v150.88,170.69 149.61,170.69 | C24.2 159.12,342.53 v159,342.65 | C28.2 158.35,140.1 v158.5,139.95 | C27.2 153.56,140.1 v153.42,139.95 | C46.2 158.86,146.95 v159,146.81 | C45.2 154.8,146.95 v154.94,146.81 | C58.2 159.4,154.57 v159.77,154.18 | C73.2 149.97,154.04 v149.86,153.92 | v146.3,152.4 C18.2 | v137.16,145.03 U29.9 | v137.16,151.38 U29.4 | v158.5,156.21 157.08,156.21 R73.1 | R71.1 v159,132.33 | C36.2 159.4,130.95 v159.51,131.06 | R56.1 v146.81,176.02 | R19.2 v151.13,176.78 | D4.3 108.13,89.22 v108.2,89.28 v109.47,89.28 | D4.7 99.24,88.58 v99.19,88.52 v97.92,88.52
  Top 0.254: v154.18,84.07 R79.1 | C32.2 157.62,54.24 v157.73,54.36 | C31.2 152.77,53.74 v152.65,53.85 | R77.1 v152.65,39.62 | R78.1 v157.73,47.75 | 154.16,49.89 v153.67,49.4 | U13.4 152.92,56.4 v152.53,56.01 | C38.2 150.73,45.1 | 150.73,45.1 v150.75,45.09 151,45.09 151.73,44.36 S6.2 | C87.2 v164.34,81.79 | C100.2 160.78,84.07 | 160.78,84.07 v161.54,84.58 | 160.78,84.07 v160.02,84.58 | C50.2 158.74,61.1 v159,60.83 | v156.08,59.94 C49.2 | U19.5 157.85,63.26 v157.86,63.25 | U19.4 153.3,63.26 v152.78,62.48 | C61.2 150.86,63.87 v150.62,63.37 | C91.2 152.16,131.97 v152.15,131.95 | v153.16,135.38 153.42,135.38 154.05,136.02 | U11.4 153.17,142.76 v152.65,142.24 | U17.4 152.41,149.62 v152.4,149.61 | U17.5 157.98,149.62 v157.99,149.61 | C83.2 v160.53,165.35 | C98.2 156.97,167.64 | 156.97,167.64 v157.73,168.4 | 156.97,167.64 v156.21,168.4 | 156.09,175.4 v156.72,176.02 | C67.1 159.12,176.26 v159.13,176.28 | D3.7 149.28,171.78 149.61,171.45 149.61,170.69 | D3.5 149.39,170.47 149.61,170.69 | R20.2 v154.69,169.93 | D3.3 140.9,171.12 v140.84,171.2 v139.57,171.2 | C2.1 113.41,181.61 v112.52,180.72 | U1.48 119.87,186.2 v120.78,186.18 | U1.5 118.88,189.75 v118.87,189.74 | U1.10 118.9,192.25 v118.87,192.28 | U1.24 113.33,193.63 v113.41,193.55 | S16.PAD 150.16,162.77 S16.1 148.38,162.77 148.08,163.07 v148.08,163.83 | C57.2 152,151.78 v152.15,151.64 | S10.2 151.51,156.97 v151.26,156.72 | v150.5,90.3 150.5,89.79 150.37,89.66 | C69.1 v154.18,89.15 | U31.9 v136.91,65.02 | C20.2 v140.72,77.98 | v149.61,73.15 150.16,72.6 S18.1 151.93,72.6 S18.PAD | C86.2 v145.8,71.88 | C75.2 v147.32,70.36 | C62.2 159.27,68.47 v159.64,68.07 | S12.2 v154.31,67.82 | C93.2 v145.54,43.94
  Top 0.254: C13.2 v106.43,184.91 | C14.2 107.39,188.65 v107.44,188.59 | C11.2 108.76,191.34 v108.84,191.26 | C12.2 108.79,193.85 v108.84,193.8 | C7.2 105.99,202.77 v105.92,202.69 | C8.2 108.89,203.28 v109.47,202.69 | C3.2 111.83,202.77 v111.76,202.69 | C4.2 114.73,202.74 v114.68,202.69 | C5.2 117.42,202.77 v117.35,202.69 | C6.2 120.32,202.77 v120.4,202.69 | R24.2 146.67,84.98 v146.69,84.71 | R23.2 146.67,93.58 v146.69,93.6 | C92.2 v32,95.76 | v32,90.68 C37.2 | R75.1 v97.79,67.31 | v96.52,59.18 C30.2 | v101.35,60.71 C29.2 | 98.95,63.65 v99.57,64.26 | v93.98,44.83 95.23,44.83 C48.2 | v99.57,44.83 100.82,44.83 C47.2 | v99.57,52.45 100.82,52.45 C59.2 | v93.98,52.45 95.23,52.45 C60.2 | v102.62,68.83 C19.2 | v111.51,71.37 U30.5 | v111.51,76.45 U30.9 | C68.1 91.81,87.77 v92.33,87.25 | C74.2 44.44,97.3 v44.32,97.41 | v94.74,92.84 96,92.84 R22.2 | R21.2 97.39,84.69 v97.41,84.71 | U12.4 99.94,49.01 v100.58,49.66 | U18.4 100.83,56.63 v100.84,56.64 | S11.2 v51.18,96.01 | C85.2 v42.42,87.12 | C99.2 44.45,90.42 | 44.45,90.42 v45.21,91.19 | v45.21,89.66 44.45,90.42 | S17.PAD 39.58,96.73 S17.1 39.58,98.51 39.88,98.81 40.39,98.81 v40.64,98.55 40.78,98.69 C84.2 v41.91,99.82 | R74.1 25.51,93.58 v25.53,93.6 | v52.83,97.28 R76.1 | D2.7 98.1,228.78 v98.04,228.73 v96.77,228.73 | R17.2 96.5,224.9 v96.52,224.92 | R18.2 96.5,232.81 v96.52,232.79 | C44.2 v100.33,234.31 | v104.9,234.31 C43.2 | v104.9,244.47 C55.2 | v100.33,244.47 C56.2 | C26.2 v101.35,254.89 | C25.2 v103.89,254.89 | v43.43,281.69 C81.2 | v32.51,282.19 33.27,282.96 | 33.27,282.96 C97.2 | 33.27,282.96 v32.51,283.72 | v59.94,282.45 C72.2 | C80.2 58.05,283.61 v57.91,283.46 | v55.12,282.19 54.57,282.74 S15.1 52.54,282.74 52.07,283.21
  Top 0.254: S15.PAD v51.56,281.69 | C35.2 96.66,268.62 v96.27,268.22 | v98.81,268.99 R68.1 | v105.66,262.38 R69.1 | R67.1 v129.54,356.62 | v102.62,317.5 C88.2 | v102.62,320.8 C33.2 | S13.1 94.04,314.25 v93.98,314.2 | S13.PAD v93.98,316.23 | C77.2 v91.95,329.18 | C95.2 95.25,330.71 | 95.25,330.71 v94.23,331.72 | 95.25,330.71 v96.27,331.72 | C22.2 94.6,346.82 v94.49,346.71 | v98.55,345.95 C21.2 | R63.1 95.11,353.46 v95,353.57 | C40.2 93.87,332.85 v93.47,333.25 | C52.2 93.61,339.71 v93.47,339.85 | C51.2 99.43,339.71 v99.57,339.85 | v98.81,304.29 R64.1 | C70.2 99.57,306.83 v98.81,306.07 | S7.2 v106.43,305.56 | v95.76,301.5 95.76,302.88 C15.2 | C94.1 v125.73,192.79 | C63.1 124.35,190.64 124.71,191.01 v125.73,191.01 | C17.2 v105.92,273.56 | U28.3 v105.92,282.7 | U28.5 v103.38,282.7 | U28.9 v98.3,282.7 | U26.9 109.65,296.6 v109.73,296.67 | U26.3 100.58,295.4 101.09,294.89 v101.85,294.89 | U26.4 v101.85,294.89 | U26.5 103.12,295.4 102.62,294.89 v101.85,294.89 | D2.5 99.72,230.65 | 99.72,230.65 v100.33,231.27 | 99.72,230.65 99.67,230.65 v99.06,231.27 | D2.1 106.47,228.13 v107.19,228.85 106.61,229.43 D2.3 | R70.1 v100.58,262.89 | U16.5 99.71,250.18 v99.57,250.32 | U16.4 105.53,250.18 v105.66,250.32 | U14.5 v93.23,344.41 v93.22,344.42 | U14.4 v99.3,344.41 v99.31,344.42 | S9.2 v65.79,285.5 | R59.1 91.31,102.62 v91.19,102.49 | R58.1 97.93,103.87 v97.79,104.01 | v116.84,85.22 R61.1 | R60.1 v116.84,93.34 | R80.1 v144.78,270.51 | C10.2 105.74,176.48 v105.54,176.28 | C9.2 v109.6,177.29 | U10.4 104.76,240.02 v105.41,240.66 | v101.09,223.52 R54.1 | R55.1 108.09,226.71 v108.2,226.82 | C76.2 93.84,310.5 v93.73,310.39 | U8.4 98.79,337.55 v99.31,338.07 | D4.5 99.61,89.88 v99.06,90.42 v97.79,90.42
  Top 0.254: D4.1 107.4,87.92 v108.2,87.12 v109.47,87.12 | D3.1 142.28,172.43 141.48,173.23 v140.72,173.23 v139.45,173.23 | R62.1 107.81,313.29 v107.7,313.18 | v157.48,362.2 157.51,362.23 C96.2 162.03,362.23 v162.05,362.2 | S8.2 151.89,350.52 v152.4,351.03 | C71.2 151.64,353.06 v152.4,352.3 | C41.2 159.65,352.92 v160.02,352.55 | C89.2 156.72,329.69 v157.48,328.93 | R65.1 161.18,327.77 161.54,327.41 v161.54,326.64 | v98.04,331.72 C39.2 | C82.2 147.69,164.23 v148.08,163.83 | v148.08,163.83 148.34,163.83 v149.1,164.59 | R72.1 v157.99,134.37 | S1.PAD 106.93,319.53 v106.17,318.77 106.17,319.79 106.64,320.26 S1.2 | S2.2 160.78,331.97 161.04,332.23 161.04,332.49 v160.53,332.99 159.77,332.23 S2.PAD | S3.2 94.48,271.53 94.74,271.27 95.5,271.27 v95.76,271.53 95.76,271.78 95,272.54 S3.PAD | S4.PAD 155.19,129.54 v155.96,130.3 156.46,129.79 156.46,129.54 156.21,129.28 S4.2 | S5.2 29.21,92.21 29.46,91.95 v30.23,91.95 30.23,92.71 29.72,93.22 S5.PAD | S6.PAD 151,44.32 150.73,44.59 150.73,45.1 | v115.57,184.91 115.82,184.91 116.33,185.42 U1.43 | C1.1 120.65,182.12 121.28,181.48 v121.28,180.85 | LED1001.C v87.12,314.71 | LED1002.C v87.12,310.64 | LED1003.C v87.12,306.58 | U27.3 151.89,315.98 v152.53,315.34 153.16,315.98 U27.4 | U27.9 160.2,316.92 v161.29,318.01 | LED1009.C v87.38,260.1 | LED1008.C v87.38,264.16 | LED1007.C v87.38,268.22 | v90.17,275.08 C90.2 | v87.38,66.04 LED1015.C | v87.38,70.36 LED1014.C | v87.38,74.42 LED1013.C | R1018.1 R1017.1 178.7,70.61 | 178.7,70.61 R1016.1 | v166.62,71.12 178.2,71.12 178.7,70.61 | R1010.1 R1011.1 178.7,116.33 | 178.7,116.33 R1012.1 | v166.62,115.95 178.32,115.95 178.7,116.33
  Top 0.508: R1006.1 R1005.1 R1004.1 178.7,316.09 177.55,317.25 167.39,317.25 v166.62,318.01
  pour Bottom: -3.81,-7.62 261.62,-7.62 261.62,384.81 -3.81,384.81
HUB_!OVRCUR1  (via drill 0.6)
  Top 0.254: U1.12 121.11,193.25 125.98,198.12 125.98,257.81 v125.6,258.19 | 130.3,345.69 125.98,341.38 125.98,338.33 v125.6,337.95 | 130.3,345.69 131.06,346.46 | 131.06,346.46 132.08,347.47 v132.08,348.23 | v135.13,348.23 135.64,348.74 v142.49,348.74 | v147.32,348.49 151.64,348.49 v153.42,350.27 | S14.5 155.91,356.4 156.46,355.85 R28.1 155.84,354.73 154.94,353.82 v154.94,351.79 | v125.6,327.02 125.98,327.41 125.98,334.77 v125.6,335.15 | v125.6,324.74 125.98,324.36 125.98,295.4 v125.6,295.02 | v125.6,292.23 125.98,291.85 125.98,260.86 v125.6,260.48 | TP33.TESTPOINT 130.3,346.46 | 130.3,346.46 130.3,345.69 | 130.3,346.46 131.06,346.46
  Bottom 0.254: v132.08,348.23 v135.13,348.23 | v142.49,348.74 147.07,348.74 v147.32,348.49 | v153.42,350.27 v154.94,351.79 | v125.6,327.02 125.98,326.64 125.98,325.12 v125.6,324.74 | v125.6,295.02 125.98,294.64 125.98,292.61 v125.6,292.23 | v125.6,260.48 125.98,260.1 125.98,258.57 v125.6,258.19 | v125.6,337.95 125.98,337.57 125.98,335.53 v125.6,335.15
HUB_!OVRCUR2  (via drill 0.6)
  Top 0.254: S13.5 97.24,319.24 v97.79,319.79 | v94.23,319.79 92.46,318.01 | 92.46,318.01 R27.1 | 92.46,318.01 v92.46,306.07 | v94.49,296.55 94.49,293.12 v97.28,290.32 | v98.81,288.8 v100.97,288.8 | v107.06,287.53 106.43,287.53 105.16,288.8 v104.01,288.8 103.89,288.67 103.89,286.51 103.38,286 TP35.TESTPOINT | v109.35,287.53 109.47,287.53 109.98,287.02 109.98,263.4 108.08,261.49 v108.08,261.11 | v108.08,257.68 108.08,257.3 108.46,256.92 108.46,241.68 v107.7,240.92 | U1.16 117.33,193.82 117.86,193.29 119.38,193.29 120.65,194.56 121.67,194.56 125.48,198.37 125.48,232.66 124.71,233.43 120.52,233.43 v120.02,233.81 | v117.73,233.81 117.35,233.43 114.81,233.43 v114.43,233.81 | v112.14,233.81 111.76,233.43 109.73,233.43 109.47,233.68 109.47,236.47 109.86,236.85 109.86,237.62 109.47,238 108.2,238 107.82,237.62 v107.7,237.62
  Bottom 0.254: v97.79,319.79 v94.23,319.79 | v92.46,306.07 92.46,304.04 94.49,302.01 v94.49,296.55 | v97.28,290.32 v98.81,288.8 | v100.97,288.8 v104.01,288.8 | v107.06,287.53 v109.35,287.53 | v108.08,261.11 v108.08,257.68 | v107.7,240.92 v107.7,237.62 | v120.02,233.81 119.63,233.43 118.11,233.43 v117.73,233.81 | v114.43,233.81 114.05,233.43 112.52,233.43 v112.14,233.81
HUB_!OVRCUR3  (via drill 0.6)
  Top 0.254: U1.20 115.33,196.84 v114.05,198.12 | v110.74,197.87 110.24,197.36 97.28,197.36 96.77,196.85 22.35,196.85 21.08,198.12 16,198.12 11.68,202.44 11.68,272.8 18.8,279.91 v36.07,279.91 | v41.15,279.91 49.02,279.91 v49.53,280.42 48.77,281.18 R29.1 | S15.5 48.55,284.69 48.39,284.86 v48.01,285.24 47.75,285.5 TP37.TESTPOINT
  Bottom 0.254: v114.05,198.12 111,198.12 v110.74,197.87 | v36.07,279.91 v41.15,279.91 | v49.53,280.42 49.53,283.72 v48.01,285.24
HUB_!OVRCUR4  (via drill 0.6)
  Top 0.254: S17.5 35.51,93.78 R31.1 35.45,94.09 34.8,94.74 30.99,94.74 v30.73,94.49 | U1.25 111.3,193.25 108.71,195.83 98.04,195.83 97.54,195.33 20.07,195.33 v19.68,195.71 | v19.68,187.83 20.07,187.45 20.07,175.51 3.81,159.26 3.81,99.06 6.22,96.65 v6.86,96.65 | v28.19,95.25 27.69,95.76 v9.91,95.76 9.91,94.74 TP39.TESTPOINT
  Bottom 0.254: v19.68,195.71 v19.68,187.83 | v6.86,96.65 9.02,96.65 v9.91,95.76 | v28.19,95.25 29.97,95.25 v30.73,94.49
HUB_!OVRCUR6  (via drill 0.6)
  Top 0.254: S18.5 154.94,70.65 v154.94,69.47 | v154.94,74.28 R32.1 152.03,74.28 151.38,74.93 151.38,77.47 151.76,77.85 v151.76,77.98 | U1.33 108.18,189.25 107.44,189.99 103.89,189.99 97.79,183.9 97.79,166.37 100.08,164.08 100.08,162.18 v100.84,161.42 | v100.84,157.1 100.58,156.84 100.58,100.33 101.09,99.82 103.5,99.82 v104.01,100.33 | v106.3,100.33 106.81,99.82 122.17,99.82 v122.56,100.2 | v126.11,100.2 v128.4,100.2 | v131.19,100.2 v134.75,100.2 | v137.54,100.2 137.79,100.2 139.06,98.93 139.19,98.81 | 139.19,98.81 141.48,96.52 141.48,90.68 v141.86,90.3 | v141.86,88.01 141.86,85.72 149.61,77.98 v149.99,77.98 | TP41.TESTPOINT 139.19,98.81
  Bottom 0.254: v154.94,69.47 v154.94,74.28 | v100.84,161.42 v100.84,157.1 | v104.01,100.33 v106.3,100.33 | v122.56,100.2 v126.11,100.2 | v128.4,100.2 v131.19,100.2 | v134.75,100.2 v137.54,100.2 | v141.86,90.3 v141.86,88.01 | v149.99,77.98 v151.76,77.98
HUB_!OVRCUR7  (via drill 0.6)
  Top 0.254: 153.12,160.82 S16.5 153.16,160.77 153.16,160.27 153.67,159.77 v153.92,159.77 | v153.92,163.83 151.64,163.83 149.86,165.61 145.8,165.61 144.53,164.34 R30.1 143.91,164.85 139.32,164.85 138.05,166.12 v137.54,166.12 | U1.37 113.33,185.72 112.78,185.17 109.98,185.17 103.89,179.07 103.89,173.48 112.01,165.61 117.35,165.61 | 117.35,165.61 118.36,165.61 | 118.36,165.61 122.94,165.61 v123.44,166.12 | v125.73,166.12 126.11,165.74 128.02,165.74 v128.4,166.12 | v130.68,166.12 131.19,165.61 134.37,165.61 v134.75,166.12 | TP43.TESTPOINT 117.86,166.12 | 117.86,166.12 117.35,165.61 | 117.86,166.12 118.36,165.61
  Bottom 0.254: v153.92,159.77 v153.92,163.83 | v123.44,166.12 v125.73,166.12 | v128.4,166.12 v130.68,166.12 | v134.75,166.12 v137.54,166.12
HUB_!PWRON1  (via drill 0.6)
  Top 0.254: U1.11 121.38,192.75 126.49,197.87 126.49,257.81 v126.87,258.19 | 130.68,345.31 126.49,341.12 126.49,338.33 v126.87,337.95 | 130.68,345.31 131.44,346.07 | v143.26,349.76 142.24,349.76 141.73,349.25 134.62,349.25 131.57,346.2 131.44,346.07 | v126.87,327.02 126.49,327.41 126.49,334.77 v126.87,335.15 | v126.87,324.74 126.49,324.36 126.49,295.4 v126.87,295.02 | v126.87,292.23 126.49,291.85 126.49,260.86 v126.87,260.48 | v146.81,349.63 147.45,349.63 148.08,349 150.11,349 150.99,349.87 S8.1 | TP32.TESTPOINT 131.44,345.31 | 131.44,345.31 130.68,345.31 | 131.44,345.31 131.44,346.07
  Bottom 0.254: v143.26,349.76 143.76,349.25 146.3,349.25 v146.81,349.63 | v126.87,327.02 126.49,326.64 126.49,325.12 v126.87,324.74 | v126.87,295.02 126.49,294.64 126.49,292.61 v126.87,292.23 | v126.87,260.48 126.49,260.1 126.49,258.57 v126.87,258.19 | v126.87,335.15 126.49,335.53 126.49,337.57 v126.87,337.95
HUB_!PWRON2  (via drill 0.6)
  Top 0.254: S7.1 105.55,304.91 105.92,304.55 v105.92,303.78 | v105.41,290.83 105.41,290.45 v107.06,288.8 | v109.35,288.8 109.47,288.8 110.49,287.78 110.49,262.25 v109.35,261.11 | v109.35,257.68 108.97,257.3 v108.97,240.92 | U1.15 117.83,194.08 118.11,193.8 119.13,193.8 120.4,195.07 121.41,195.07 124.97,198.63 124.97,232.41 124.46,232.92 120.4,232.92 v120.02,232.54 | v117.73,232.54 117.35,232.92 114.81,232.92 v114.43,232.54 | v112.14,232.54 111.76,232.92 109.47,232.92 108.97,233.43 v108.97,237.11
  Bottom 0.254: v105.92,303.78 105.92,293.37 105.41,292.86 v105.41,290.83 | v109.35,288.8 v107.06,288.8 106.17,287.91 106.17,286.77 106.43,286.51 TP34.TESTPOINT | v109.35,261.11 v109.35,257.68 | v108.97,240.92 v108.97,237.11 | v120.02,232.54 119.63,232.92 118.11,232.92 v117.73,232.54 | v114.43,232.54 114.05,232.92 112.52,232.92 v112.14,232.54
HUB_!PWRON3  (via drill 0.6)
  Top 0.254: U1.19 115.83,197.61 v115.32,198.12 | v111.76,197.23 111.38,196.85 97.54,196.85 97.03,196.34 22.1,196.34 20.83,197.61 15.75,197.61 11.18,202.18 11.18,273.05 24.89,286.77 51.82,286.77 v52.32,286.26 | 64.77,284.73 v65.02,284.48 64.66,284.85 S9.1
  Bottom 0.254: v115.32,198.12 114.3,196.85 112.14,196.85 v111.76,197.23 | v52.32,286.26 52.83,286.77 58.17,286.77 58.55,287.15 59.31,287.15 61.72,284.73 64.77,284.73 v65.02,284.48 TP36.TESTPOINT
HUB_!PWRON4  (via drill 0.6)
